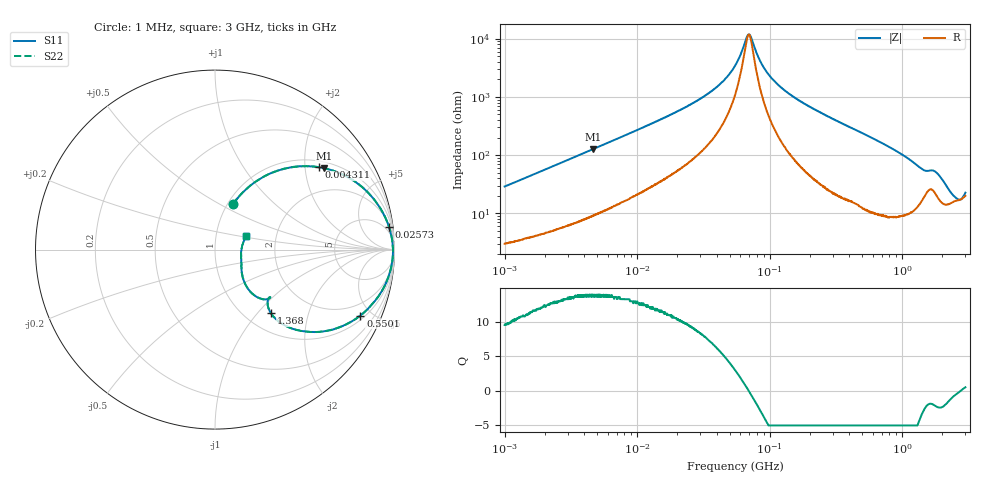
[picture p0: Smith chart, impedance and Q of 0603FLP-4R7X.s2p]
!s-Parameter Generated by FASTRON Sdn. Bhd.
!FASTRON P/N : 0603FLP-4R7X
!Keysight Technologies: E4991B_MY54100416_A.01.15
!Date: Tue Dec 02 13:04:26 2025
!Version  :Rev00  Tue Dec 02 13:04:26 2025
!Data & Calibration Information:
!Freq  S11  S21  S12  S22
!PortZ  Port1:50+j0  Port2:50+j0
!When reading reference impedance value at option line is always used.
! Remarks : This data is being provided solely for informational purposes.
# Hz S dB R 50
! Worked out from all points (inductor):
!   1601 points, 1 MHz to 3 GHz, reference 50 ohm
!   read as one part in series: L = 4.52 uH near 1.041 MHz
!   highest Q = 13.9 at 4.624 MHz (marker M1), where L = 4.34 uH
!   self-resonance near 69.67 MHz
!   S11 on the Smith chart (normalised r, x): 1 MHz: 1.06, +0.58; 4.311 MHz: 1.17, +2.36; 25.73 MHz: 3, +15; 550.1 MHz: 1.22, -4.29; 1.368 GHz: 1.30, -1.18; 3 GHz: 1.40, +0.21
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1000000  -11.30 68.4  -0.59 -15.6  -0.59 -15.6  -11.30 68.4
1916532  -6.77 58.1  -1.40 -27.2  -1.40 -27.2  -6.77 58.1
3804036  -3.13 41.8  -3.51 -44.1  -3.51 -44.1  -3.13 41.8
4310966  -2.65 38.5  -4.09 -47.3  -4.09 -47.3  -2.65 38.5
4623804  -2.41 36.8  -4.44 -49.1  -4.44 -49.1  -2.41 36.8
1.447069e7  -0.44 13.9  -12.40 -71.2  -12.40 -71.2  -0.44 13.9
2.572808e7  -0.19 7.4  -17.80 -76.5  -17.80 -76.5  -0.19 7.4
4.05666e7  -0.11 3.6  -23.80 -77.0  -23.80 -77.0  -0.11 3.6
5.504702e7  -0.08 1.6  -30.90 -69.9  -30.90 -69.9  -0.08 1.6
6.690963e7  -0.07 0.3  -40.30 -28.4  -40.30 -28.4  -0.07 0.3
7.034296e7  -0.07 -0.1  -41.50 7.7  -41.50 7.7  -0.07 -0.1
8.550185e7  -0.07 -1.4  -32.10 69.9  -32.10 69.9  -0.07 -1.4
1.02379e8  -0.08 -2.6  -26.80 77.4  -26.80 77.4  -0.08 -2.6
1.361705e8  -0.10 -4.7  -21.60 79.6  -21.60 79.6  -0.10 -4.7
2.083556e8  -0.19 -8.7  -16.40 77.6  -16.40 77.6  -0.19 -8.7
5.500551e8  -1.02 -24.4  -7.66 62.6  -7.66 62.6  -1.02 -24.4
7.925923e8  -2.05 -34.4  -4.94 52.1  -4.94 52.1  -2.05 -34.4
1.075512e9  -3.82 -44.2  -3.09 39.9  -3.09 39.9  -3.82 -44.2
1.367504e9  -6.54 -48.7  -2.22 27.2  -2.22 27.2  -6.54 -48.7
1.86495e9  -8.53 -46.9  -2.01 20.2  -2.01 20.2  -8.53 -46.9
2.620866e9  -16.40 -15.5  -1.36 2.7  -1.36 2.7  -16.40 -15.5
3e9  -14.50 22.9  -1.62 -5.1  -1.62 -5.1  -14.50 22.9
